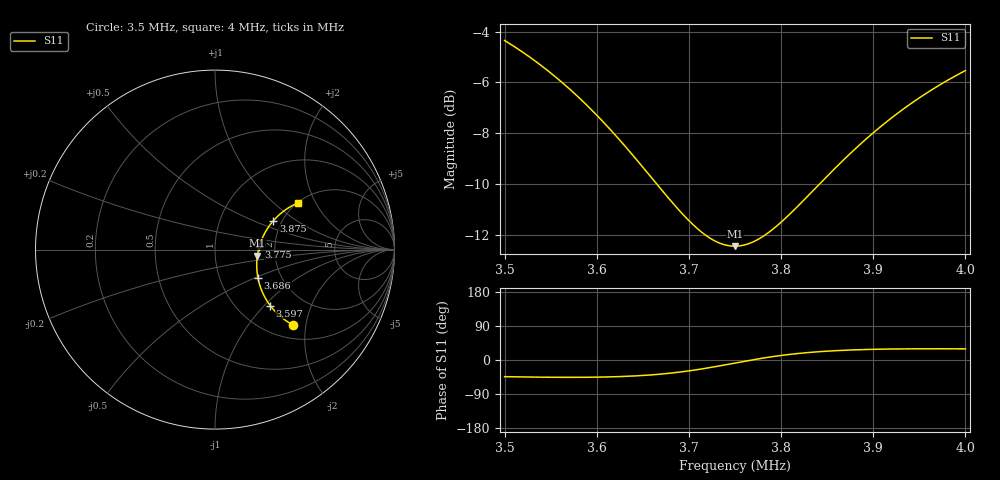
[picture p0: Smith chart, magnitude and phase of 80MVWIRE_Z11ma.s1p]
# MHz Z MA R 50
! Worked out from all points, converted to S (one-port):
!   501 points, 3.5 MHz to 4 MHz, reference 50 ohm
!   lowest |S11| = -12.4 dB at 3.75 MHz (marker M1), VSWR 1.63, Z = 80.7 - j5.65 ohm
!   |S11| at or under -10 dB: 3.665 MHz to 3.842 MHz (176.6 kHz wide, 4.71 % of centre)
!   S11 on the Smith chart (normalised r, x): 3.5 MHz: 1.28, -1.70; 3.597 MHz: 1.40, -1.08; 3.686 MHz: 1.52, -0.52; 3.775 MHz: 1.65, +0.04; 3.875 MHz: 1.80, +0.67; 4 MHz: 2.01, +1.45
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3.5  2.128 -53.1
3.514  2.068 -51.2
3.531  1.998 -48.8
3.547  1.936 -46.3
3.563  1.878 -43.7
3.58  1.821 -40.7
3.597  1.77 -37.6
3.625  1.698 -32.1
3.641  1.666 -28.7
3.656  1.64 -25.5
3.671  1.621 -22.1
3.686  1.607 -18.7
3.688  1.606 -18.3
3.706  1.599 -14.1
3.722  1.6 -10.4
3.736  1.606 -7.2
3.743  1.611 -5.6
3.75  1.618 -4.0
3.762  1.632 -1.3
3.775  1.651 1.5
3.792  1.683 5.1
3.813  1.731 9.4
3.844  1.819 15.2
3.875  1.925 20.4
3.906  2.045 25.0
3.938  2.183 29.1
3.97  2.332 32.8
4  2.48 35.8
